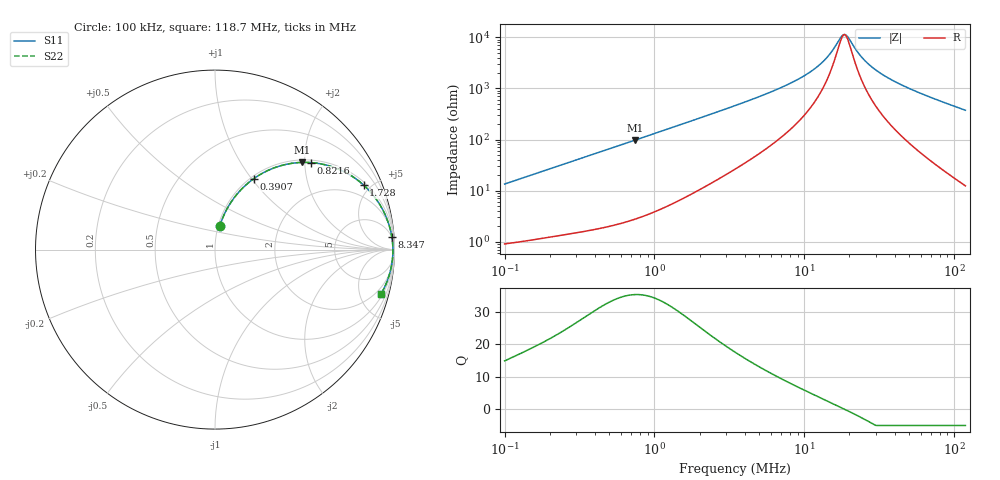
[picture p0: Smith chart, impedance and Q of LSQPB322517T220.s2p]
! LSQPB322517T220  S-PARAMETER MODEL  ( General Type )
! Model Generated by TAIYO YUDEN Corporation (http://www.ty-top.com)
! Version 2.0
! TAIYO YUDEN Control No. 100810NC14SB-FKC
! Copyright(c) 2008 TAIYO YUDEN CO.,LTD. All Rights Reserved.
! Product Description (link to TY-COMPAS)
! https://ds.yuden.co.jp/TYCOMPAS/or/detail?pn=LSQPB322517T220K&u=M
! Products Name : Inductors
! Characteristics :
!  Inductance : 22 uH , SRF(min) : 13 MHz , DC Resistance(max) : 0.828 Ohm
!  Rated Current : Saturation :550 mA , Temp Rise : 470 mA (40 degC)
!  Case Size : 3.2 x 2.5 / 0.126 x 0.098 [mm/inch] , Thickness : 1.7 / 0.068 [mm/inch]
!  (Conditions: Temperature = 25 degC , DC Bias Current/Voltage = 0A / 0V)
! External Node Assignments :
!  1  o---GGG---o  2
! GND o---------o GND
! Frequency Range : 0.1MHz  -  118.695536MHz  [ 402 STEP ]
# MHz S RI R 50
! Freq[MHz].  S11 Real  S11 Imag  S21 Real  S21 Imag  S12 Real  S12 Imag  S22 Real  S22 Imag
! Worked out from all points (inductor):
!   401 points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, 100 kHz to 118.7 MHz, reference 50 ohm
!   read as one part in series: L = 21.3 uH near 103.6 kHz
!   highest Q = 35.2 at 738.8 kHz (marker M1), where L = 20.8 uH
!   self-resonance near 18.18 MHz
!   S11 on the Smith chart (normalised r, x): 100 kHz: 1.02, +0.27; 390.7 kHz: 1.03, +1.03; 821.6 kHz: 1.06, +2.15; 1.728 MHz: 1.17, +4.53; 8.347 MHz: 4, +26; 118.7 MHz: 1.25, -7.48
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0.1  0.0261 0.1294  0.9739 -0.1294  0.9739 -0.1294  0.0261 0.1294
0.195917  0.0731 0.2381  0.9269 -0.2381  0.9269 -0.2381  0.0731 0.2381
0.327316  0.1657 0.3542  0.8343 -0.3542  0.8343 -0.3542  0.1657 0.3542
0.390687  0.2166 0.3956  0.7834 -0.3956  0.7834 -0.3956  0.2166 0.3956
0.738801  0.4842 0.4858  0.5158 -0.4858  0.5158 -0.4858  0.4842 0.4858
0.821569  0.5357 0.4847  0.4643 -0.4847  0.4643 -0.4847  0.5357 0.4847
1.07136  0.6588 0.4595  0.3412 -0.4595  0.3412 -0.4595  0.6588 0.4595
1.727666  0.8283 0.3593  0.1717 -0.3593  0.1717 -0.3593  0.8283 0.3593
3.445222  0.9445 0.2022  0.0555 -0.2022  0.0555 -0.2022  0.9445 0.2022
5.755906  0.9752 0.1179  0.0248 -0.1179  0.0248 -0.1179  0.9752 0.1179
8.346829  0.9849 0.0728  0.0151 -0.0728  0.0151 -0.0728  0.9849 0.0728
11.27678  0.9889 0.0428  0.0111 -0.0428  0.0111 -0.0428  0.9889 0.0428
13.94498  0.9905 0.0239  0.00952 -0.0239  0.00952 -0.0239  0.9905 0.0239
17.55242  0.9912 0.00442  0.00875 -0.00442  0.00875 -0.00442  0.9912 0.00442
18.50953  0.9913 -2.12e-05  0.00869 2.12e-05  0.00869 2.12e-05  0.9913 -2.12e-05
19.51882  0.9913 -0.00446  0.00867 0.00446  0.00867 0.00446  0.9913 -0.00446
22.88908  0.9911 -0.0179  0.00888 0.0179  0.00888 0.0179  0.9911 -0.0179
25.90783  0.9907 -0.0287  0.00934 0.0287  0.00934 0.0287  0.9907 -0.0287
30.38126  0.9897 -0.0432  0.0103 0.0432  0.0103 0.0432  0.9897 -0.0432
36.91074  0.9877 -0.0623  0.0123 0.0623  0.0123 0.0623  0.9877 -0.0623
60.58472  0.9762 -0.1226  0.0238 0.1226  0.0238 0.1226  0.9762 -0.1226
118.6955  0.9264 -0.2452  0.0736 0.2452  0.0736 0.2452  0.9264 -0.2452
